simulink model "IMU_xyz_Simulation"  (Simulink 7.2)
settings: Solver=FixedStepDiscrete  StartTime=0.0  StopTime=110  FixedStep=.001  RelTol=1e-3
PreLoadFcn:
  | Script_Kalman
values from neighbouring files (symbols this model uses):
  Az = [1 -Ts ;0 1]    [Script_Kalman.m]
  Kz = 1e-3*[.4 ; -.04]    [Script_Kalman.m]
  Ts = .001    (= 0.001)    [Script_Kalman.m]
undefined symbols (not defined in the file or in its folder): DiscIntNeverNeededParam, float
libraries: simulink x40
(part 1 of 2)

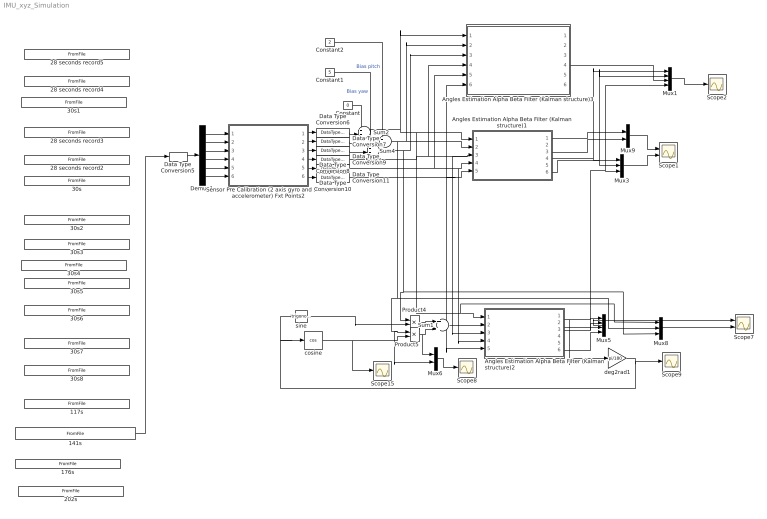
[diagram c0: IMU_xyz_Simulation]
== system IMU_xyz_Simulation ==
  117s : FromFile  FileName=LongLogHorizontalSmallRoll.mat  SampleTime=.001
  141s : FromFile  FileName=LongLongLogHorizontalSmallRoll.mat  SampleTime=.001
  176s : FromFile  FileName=LongLongLogHorizontalSmallRoll2.mat  SampleTime=.001
  202s : FromFile  FileName=LongLongLogHorizontalStatic.mat  SampleTime=.001
  28 seconds record2 : FromFile  FileName=Pitch.mat  SampleTime=.001
  28 seconds record3 : FromFile  FileName=Yaw.mat  SampleTime=.001
  28 seconds record4 : FromFile  FileName=Pitch2.mat  SampleTime=.001
  28 seconds record5 : FromFile  FileName=Yaw2.mat  SampleTime=.001
  30s : FromFile  FileName=Roll.mat  SampleTime=.001
  30s1 : FromFile  FileName=Roll2.mat  SampleTime=.001
  30s2 : FromFile  FileName=Pitch_Up_Calibration.mat  SampleTime=.001
  30s3 : FromFile  FileName=Roll_Right_Calibration.mat  SampleTime=.001
  30s4 : FromFile  FileName=Turn_Left_Roll_Pitch_Yaw.mat  SampleTime=.001
  30s5 : FromFile  FileName=Turn_Left_Right_Roll_Pitch_Yaw.mat  SampleTime=.001
  30s6 : FromFile  FileName=Turn_Left_Right.mat  SampleTime=.001
  30s7 : FromFile  FileName=StaticHorizontal.mat  SampleTime=.001
  30s8 : FromFile  FileName=StaticRoll90.mat  SampleTime=.001
  Angles Estimation Alpha Beta Filter (Kalman structure)1 : Subsystem
  Angles Estimation Alpha Beta Filter (Kalman structure)2 : Subsystem
  Angles Estimation Alpha Beta Filter (Kalman structure)3 : Subsystem
  Constant : Constant  Value=0  OutDataType=sfix(16)  OutScaling=2^0
  Constant1 : Constant  Value=5  OutDataType=sfix(16)  OutScaling=2^0
  Constant2 : Constant  Value=2  OutDataType=sfix(16)  OutScaling=2^0
  Data Type Conversion{6..11} (6 alike) : DataTypeConversion  OutDataType=sfix(16)  OutScaling=2^0
  Data Type Conversion5 : DataTypeConversion  OutDataTypeMode=int16  OutDataType=sfix(16)  OutScaling=2^0  OutDataTypeStr=int16
  Demux1 : Demux  Outputs=6
  Mux1 : Mux
  Mux3 : Mux  Inputs=3
  Mux5 : Mux
  Mux6 : Mux  Inputs=2
  Mux8 : Mux  Inputs=3
  Mux9 : Mux  Inputs=2
  Product4 : Product  OutDataType=sfix(16)  OutScaling=2^0
  Product5 : Product  OutDataType=sfix(16)  OutScaling=2^0
  Scope1 : Scope  NumInputPorts=2
  Scope{2,8..9,15} (4 alike) : Scope
  Scope7 : Scope  NumInputPorts=2
  Sensor Pre Calibration (2 axis gyro and 3 axis accelerometer) Fxt Points2 : Subsystem
  Sum1 : Sum  OutDataType=sfix(16)  OutScaling=2^0
  Sum2 : Sum  Inputs=++|  OutDataType=sfix(16)  OutScaling=2^0
  Sum3 : Sum  Inputs=++|  OutDataType=sfix(16)  OutScaling=2^0
  Sum4 : Sum  Inputs=++|  OutDataType=sfix(16)  OutScaling=2^0
  cosine : Trigonometry  Operator=cos
  deg2rad1 : Gain  Gain=pi/180  ParameterDataType=sfix(16)  ParameterScaling=2^0  OutDataType=sfix(16)  OutScaling=2^0
  sine : Trigonometry
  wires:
  Demux1/1 -> Sensor Pre Calibration (2 axis gyro and 3 axis accelerometer) Fxt Points2/1(Gyro Y)
  Demux1/2 -> Sensor Pre Calibration (2 axis gyro and 3 axis accelerometer) Fxt Points2/2(Accel y)
  Demux1/3 -> Sensor Pre Calibration (2 axis gyro and 3 axis accelerometer) Fxt Points2/3(Accel z)
  Demux1/4 -> Sensor Pre Calibration (2 axis gyro and 3 axis accelerometer) Fxt Points2/4(Gyro X)
  Demux1/5 -> Sensor Pre Calibration (2 axis gyro and 3 axis accelerometer) Fxt Points2/5(Accel x)
  Demux1/6 -> Sensor Pre Calibration (2 axis gyro and 3 axis accelerometer) Fxt Points2/6(Gyro z)
  Data Type Conversion5/1 -> Demux1/1
  Sensor Pre Calibration (2 axis gyro and 3 axis accelerometer) Fxt Points2/6(unbiased Accel Z) -> Data Type Conversion11/1
  Sensor Pre Calibration (2 axis gyro and 3 axis accelerometer) Fxt Points2/1(Gyro Y (degree/s)) -> Data Type Conversion6/1
  Sensor Pre Calibration (2 axis gyro and 3 axis accelerometer) Fxt Points2/2(Gyro X (degree/s)) -> Data Type Conversion7/1
  Sensor Pre Calibration (2 axis gyro and 3 axis accelerometer) Fxt Points2/3(Gyro Z (degree/s)) -> Data Type Conversion8/1
  Data Type Conversion6/1 -> Sum2/2
  Data Type Conversion7/1 -> Sum4/2
  Sensor Pre Calibration (2 axis gyro and 3 axis accelerometer) Fxt Points2/4(unbiased Accel Y) -> Data Type Conversion9/1
  Sensor Pre Calibration (2 axis gyro and 3 axis accelerometer) Fxt Points2/5(unbiased Accel X) -> Data Type Conversion10/1
  Data Type Conversion9/1 -> Angles Estimation Alpha Beta Filter (Kalman structure)3/4(Accel Y), Angles Estimation Alpha Beta Filter (Kalman structure)1/3(Accel Y), Angles Estimation Alpha Beta Filter (Kalman structure)2/3(Accel Y)
  Data Type Conversion10/1 -> Angles Estimation Alpha Beta Filter (Kalman structure)1/4(Accel X), Angles Estimation Alpha Beta Filter (Kalman structure)2/4(Accel X), Angles Estimation Alpha Beta Filter (Kalman structure)3/5(Accel X)
  Data Type Conversion11/1 -> Angles Estimation Alpha Beta Filter (Kalman structure)1/5(Accel Z), Angles Estimation Alpha Beta Filter (Kalman structure)2/5(Accel Z), Angles Estimation Alpha Beta Filter (Kalman structure)3/6(Accel Z)
  Data Type Conversion8/1 -> Sum3/2
  Mux5/1 -> Scope7/1
  Angles Estimation Alpha Beta Filter (Kalman structure)2/1(Angle Estimation Y) -> deg2rad1/1, Mux5/1
  Angles Estimation Alpha Beta Filter (Kalman structure)2/4(Angle Estimation X) -> Mux5/2, Mux3/3, Mux1/4
  deg2rad1/1 -> sine/1, cosine/1, Scope9/1
  cosine/1 -> Product5/2, Scope15/1
  Sum1/1 -> Angles Estimation Alpha Beta Filter (Kalman structure)2/2(Gyro X)
  Product5/1 -> Sum1/2, Mux6/1
  Product4/1 -> Sum1/1
  sine/1 -> Product4/2
  Mux6/1 -> Scope8/1
  Mux8/1 -> Scope7/2
  Angles Estimation Alpha Beta Filter (Kalman structure)2/3(Angle Estimation Y Accel) -> Mux5/3
  Angles Estimation Alpha Beta Filter (Kalman structure)2/6(Angle Estimation X  Accel) -> Mux5/4
  Angles Estimation Alpha Beta Filter (Kalman structure)1/1(Angle Estimation Y) -> Mux9/1
  Angles Estimation Alpha Beta Filter (Kalman structure)1/3(Angle Estimation Y Accel) -> Mux9/2
  Angles Estimation Alpha Beta Filter (Kalman structure)1/4(Angle Estimation X) -> Mux3/1, Mux1/1
  Angles Estimation Alpha Beta Filter (Kalman structure)1/6(Angle Estimation X  Accel) -> Mux3/2, Mux1/2
  Mux9/1 -> Scope1/1
  Mux3/1 -> Scope1/2
  Angles Estimation Alpha Beta Filter (Kalman structure)3/4(Angle Estimation X) -> Mux1/3
  Mux1/1 -> Scope2/1
  Sum2/1 -> Angles Estimation Alpha Beta Filter (Kalman structure)2/1(Gyro Y), Mux8/1, Angles Estimation Alpha Beta Filter (Kalman structure)1/1(Gyro Y), Angles Estimation Alpha Beta Filter (Kalman structure)3/1(Gyro Y)
  Constant/1 -> Sum2/1
  Sum3/1 -> Angles Estimation Alpha Beta Filter (Kalman structure)3/3(Gyro Z), Product4/1, Mux8/3
  Constant1/1 -> Sum3/1  "Bias yaw"
  Sum4/1 -> Product5/1, Mux6/2, Mux8/2, Angles Estimation Alpha Beta Filter (Kalman structure)3/2(Gyro X), Angles Estimation Alpha Beta Filter (Kalman structure)1/2(Gyro X)
  Constant2/1 -> Sum4/1  "Bias pitch"
  141s/1 -> Data Type Conversion5/1

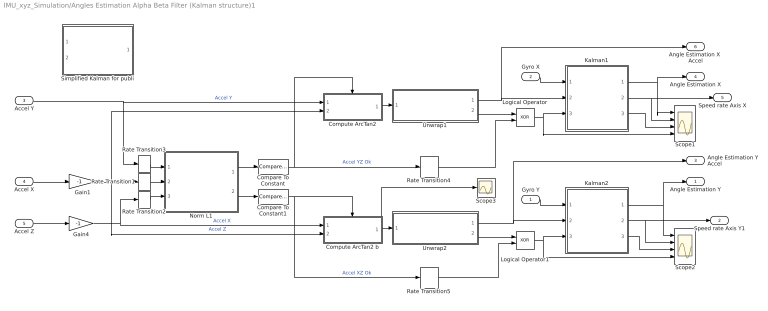
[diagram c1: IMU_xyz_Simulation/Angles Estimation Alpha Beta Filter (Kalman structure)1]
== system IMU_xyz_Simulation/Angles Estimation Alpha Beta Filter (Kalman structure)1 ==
  Gyro Y : Inport
  Gyro X : Inport  Port=2
  Accel Y : Inport  Port=3
  Accel X : Inport  Port=4
  Accel Z : Inport  Port=5
  Compare To Constant : simulink/Logic and Bit Operations/Compare To Constant  SystemSampleTime=-1  relop=>=  const=200  LogicOutDataTypeMode=boolean  ZeroCross=off
  Compare To Constant1 : simulink/Logic and Bit Operations/Compare To Constant  SystemSampleTime=-1  relop=>=  const=200  LogicOutDataTypeMode=boolean  ZeroCross=off
  Compute ArcTan2 : Subsystem
  Compute ArcTan2 b : Subsystem
  Gain1 : Gain  Gain=-1  ParameterDataType=sfix(16)  ParameterScaling=2^0  OutDataType=sfix(16)  OutScaling=2^0
  Gain4 : Gain  Gain=-1  ParameterDataType=sfix(16)  ParameterScaling=2^0  OutDataType=sfix(16)  OutScaling=2^0
  Kalman1 : Subsystem
  Kalman2 : Subsystem
  Logical Operator : Logic  Operator=XOR  AllPortsSameDT=off  OutDataTypeMode=boolean  OutDataTypeStr=boolean
  Logical Operator1 : Logic  Operator=XOR  AllPortsSameDT=off  OutDataTypeMode=boolean  OutDataTypeStr=boolean
  Norm L1 : Subsystem
  Rate Transition1 : RateTransition  Integrity=off  OutPortSampleTime=.2
  Rate Transition2 : RateTransition  Integrity=off  OutPortSampleTime=.2
  Rate Transition3 : RateTransition  Integrity=off  OutPortSampleTime=.2
  Rate Transition4 : RateTransition  Integrity=off  OutPortSampleTime=.001
  Rate Transition5 : RateTransition  Integrity=off  OutPortSampleTime=.001
  Scope1 : Scope  NumInputPorts=4
  Scope2 : Scope  NumInputPorts=4
  Scope3 : Scope
  Simplified Kalman for publi : Subsystem
  Unwrap1 : Subsystem
  Unwrap2 : Subsystem
  Angle Estimation Y : Outport
  Speed rate Axis Y1 : Outport  Port=2
  Angle Estimation Y Accel : Outport  Port=3
  Angle Estimation X : Outport  Port=4
  Speed rate Axis X : Outport  Port=5
  Angle Estimation X  Accel : Outport  Port=6
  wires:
  Kalman1/3(Bias) -> Scope1/3
  Kalman2/3(Bias) -> Scope2/3
  Kalman2/2(Speed) -> Speed rate Axis Y1/1, Scope2/2
  Kalman1/2(Speed) -> Speed rate Axis X/1, Scope1/2
  Unwrap2/1(unwrap angle) -> Angle Estimation Y Accel/1, Kalman2/2(Accel1)
  Unwrap2/2(Wrap) -> Logical Operator1/1
  Logical Operator/1 -> Scope1/4, Kalman1/3(Adapt1)
  Rate Transition5/1 -> Logical Operator1/2
  Gain1/1 -> Compute ArcTan2 b/2(Force 2), Rate Transition1/1, Compute ArcTan2/2(Force 2)  "Accel Z"
  Logical Operator1/1 -> Kalman2/3(Adapt1), Scope2/4
  Rate Transition4/1 -> Logical Operator/2
  Unwrap1/2(Wrap) -> Logical Operator/1
  Unwrap1/1(unwrap angle) -> Angle Estimation X  Accel/1, Kalman1/2(Accel1)
  Rate Transition3/1 -> Norm L1/1(Accel Y)
  Rate Transition2/1 -> Norm L1/3(Accel X)
  Rate Transition1/1 -> Norm L1/2(Accel Z)
  Kalman2/1(Position) -> Scope2/1, Angle Estimation Y/1
  Kalman1/1(Position) -> Scope1/1, Angle Estimation X/1
  Compare To Constant1/1 -> Rate Transition5/1, Compute ArcTan2 b/Enable  "Accel XZ Ok"
  Compare To Constant/1 -> Rate Transition4/1, Compute ArcTan2/Enable  "Accel YZ Ok"
  Norm L1/1(abs(Y)+abs(Z)) -> Compare To Constant/1
  Norm L1/2(abs(X)+abs(Z)) -> Compare To Constant1/1
  Accel X/1 -> Gain1/1
  Gain4/1 -> Compute ArcTan2 b/1(Force 1), Rate Transition2/1  "Accel X"
  Compute ArcTan2/1(Degree) -> Unwrap1/1(Estimated Angle)
  Compute ArcTan2 b/1(Degree) -> Scope3/1, Unwrap2/1(Estimated Angle)
  Accel Z/1 -> Gain4/1
  Accel Y/1 -> Compute ArcTan2/1(Force 1), Rate Transition3/1  "Accel Y"
  Gyro X/1 -> Kalman1/1(Gyro)
  Gyro Y/1 -> Kalman2/1(Gyro)

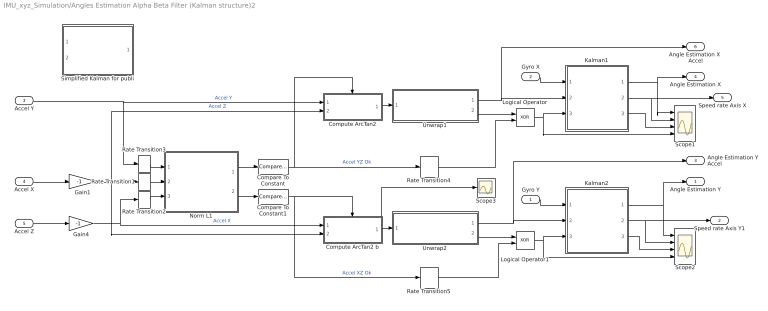
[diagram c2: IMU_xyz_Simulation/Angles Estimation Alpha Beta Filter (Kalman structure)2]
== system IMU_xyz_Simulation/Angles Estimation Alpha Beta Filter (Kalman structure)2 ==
  Gyro Y : Inport
  Gyro X : Inport  Port=2
  Accel Y : Inport  Port=3
  Accel X : Inport  Port=4
  Accel Z : Inport  Port=5
  Compare To Constant : simulink/Logic and Bit Operations/Compare To Constant  SystemSampleTime=-1  relop=>=  const=200  LogicOutDataTypeMode=boolean  ZeroCross=off
  Compare To Constant1 : simulink/Logic and Bit Operations/Compare To Constant  SystemSampleTime=-1  relop=>=  const=200  LogicOutDataTypeMode=boolean  ZeroCross=off
  Compute ArcTan2 : Subsystem
  Compute ArcTan2 b : Subsystem
  Gain1 : Gain  Gain=-1  ParameterDataType=sfix(16)  ParameterScaling=2^0  OutDataType=sfix(16)  OutScaling=2^0
  Gain4 : Gain  Gain=-1  ParameterDataType=sfix(16)  ParameterScaling=2^0  OutDataType=sfix(16)  OutScaling=2^0
  Kalman1 : Subsystem
  Kalman2 : Subsystem
  Logical Operator : Logic  Operator=XOR  AllPortsSameDT=off  OutDataTypeMode=boolean  OutDataTypeStr=boolean
  Logical Operator1 : Logic  Operator=XOR  AllPortsSameDT=off  OutDataTypeMode=boolean  OutDataTypeStr=boolean
  Norm L1 : Subsystem
  Rate Transition1 : RateTransition  Integrity=off  OutPortSampleTime=.2
  Rate Transition2 : RateTransition  Integrity=off  OutPortSampleTime=.2
  Rate Transition3 : RateTransition  Integrity=off  OutPortSampleTime=.2
  Rate Transition4 : RateTransition  Integrity=off  OutPortSampleTime=.001
  Rate Transition5 : RateTransition  Integrity=off  OutPortSampleTime=.001
  Scope1 : Scope  NumInputPorts=4
  Scope2 : Scope  NumInputPorts=4
  Scope3 : Scope
  Simplified Kalman for publi : Subsystem
  Unwrap1 : Subsystem
  Unwrap2 : Subsystem
  Angle Estimation Y : Outport
  Speed rate Axis Y1 : Outport  Port=2
  Angle Estimation Y Accel : Outport  Port=3
  Angle Estimation X : Outport  Port=4
  Speed rate Axis X : Outport  Port=5
  Angle Estimation X  Accel : Outport  Port=6
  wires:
  Gyro Y/1 -> Kalman2/1(Gyro)
  Gyro X/1 -> Kalman1/1(Gyro)
  Accel Y/1 -> Rate Transition3/1, Compute ArcTan2/1(Force 1)  "Accel Y"
  Accel Z/1 -> Gain4/1
  Compute ArcTan2 b/1(Degree) -> Unwrap2/1(Estimated Angle), Scope3/1
  Compute ArcTan2/1(Degree) -> Unwrap1/1(Estimated Angle)
  Gain4/1 -> Rate Transition2/1, Compute ArcTan2 b/1(Force 1)  "Accel X"
  Accel X/1 -> Gain1/1
  Norm L1/2(abs(X)+abs(Z)) -> Compare To Constant1/1
  Norm L1/1(abs(Y)+abs(Z)) -> Compare To Constant/1
  Compare To Constant/1 -> Compute ArcTan2/Enable, Rate Transition4/1  "Accel YZ Ok"
  Compare To Constant1/1 -> Compute ArcTan2 b/Enable, Rate Transition5/1  "Accel XZ Ok"
  Kalman1/1(Position) -> Angle Estimation X/1, Scope1/1
  Kalman2/1(Position) -> Angle Estimation Y/1, Scope2/1
  Rate Transition1/1 -> Norm L1/2(Accel Z)
  Rate Transition2/1 -> Norm L1/3(Accel X)
  Rate Transition3/1 -> Norm L1/1(Accel Y)
  Unwrap1/1(unwrap angle) -> Kalman1/2(Accel1), Angle Estimation X  Accel/1
  Unwrap1/2(Wrap) -> Logical Operator/1
  Rate Transition4/1 -> Logical Operator/2
  Logical Operator1/1 -> Scope2/4, Kalman2/3(Adapt1)
  Gain1/1 -> Compute ArcTan2/2(Force 2), Rate Transition1/1, Compute ArcTan2 b/2(Force 2)  "Accel Z"
  Rate Transition5/1 -> Logical Operator1/2
  Logical Operator/1 -> Kalman1/3(Adapt1), Scope1/4
  Unwrap2/2(Wrap) -> Logical Operator1/1
  Unwrap2/1(unwrap angle) -> Kalman2/2(Accel1), Angle Estimation Y Accel/1
  Kalman1/2(Speed) -> Scope1/2, Speed rate Axis X/1
  Kalman2/2(Speed) -> Scope2/2, Speed rate Axis Y1/1
  Kalman2/3(Bias) -> Scope2/3
  Kalman1/3(Bias) -> Scope1/3

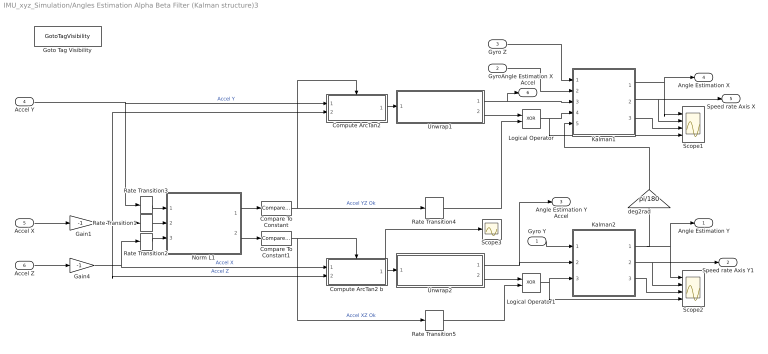
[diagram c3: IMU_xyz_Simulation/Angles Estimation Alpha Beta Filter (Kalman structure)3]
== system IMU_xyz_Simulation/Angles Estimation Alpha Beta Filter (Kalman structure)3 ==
  Gyro Y : Inport
  Gyro X : Inport  Port=2
  Gyro Z : Inport  Port=3
  Accel Y : Inport  Port=4
  Accel X : Inport  Port=5
  Accel Z : Inport  Port=6
  Compare To Constant : simulink/Logic and Bit Operations/Compare To Constant  SystemSampleTime=-1  relop=>=  const=200  LogicOutDataTypeMode=boolean  ZeroCross=off
  Compare To Constant1 : simulink/Logic and Bit Operations/Compare To Constant  SystemSampleTime=-1  relop=>=  const=200  LogicOutDataTypeMode=boolean  ZeroCross=off
  Compute ArcTan2 : Subsystem
  Compute ArcTan2 b : Subsystem
  Gain1 : Gain  Gain=-1  ParameterDataType=sfix(16)  ParameterScaling=2^0  OutDataType=sfix(16)  OutScaling=2^0
  Gain4 : Gain  Gain=-1  ParameterDataType=sfix(16)  ParameterScaling=2^0  OutDataType=sfix(16)  OutScaling=2^0
  Goto Tag Visibility : GotoTagVisibility
  Kalman1 : Subsystem
  Kalman2 : Subsystem
  Logical Operator : Logic  Operator=XOR  AllPortsSameDT=off  OutDataTypeMode=boolean  OutDataTypeStr=boolean
  Logical Operator1 : Logic  Operator=XOR  AllPortsSameDT=off  OutDataTypeMode=boolean  OutDataTypeStr=boolean
  Norm L1 : Subsystem
  Rate Transition1 : RateTransition  Integrity=off  OutPortSampleTime=.2
  Rate Transition2 : RateTransition  Integrity=off  OutPortSampleTime=.2
  Rate Transition3 : RateTransition  Integrity=off  OutPortSampleTime=.2
  Rate Transition4 : RateTransition  Integrity=off  OutPortSampleTime=.001
  Rate Transition5 : RateTransition  Integrity=off  OutPortSampleTime=.001
  Scope1 : Scope  NumInputPorts=4
  Scope2 : Scope  NumInputPorts=4
  Scope3 : Scope
  Unwrap1 : Subsystem
  Unwrap2 : Subsystem
  deg2rad : Gain  Orientation=up  Gain=pi/180  ParameterDataType=sfix(16)  ParameterScaling=2^0  OutDataType=sfix(16)  OutScaling=2^0
  Angle Estimation Y : Outport
  Speed rate Axis Y1 : Outport  Port=2
  Angle Estimation Y Accel : Outport  Port=3
  Angle Estimation X : Outport  Port=4
  Speed rate Axis X : Outport  Port=5
  Angle Estimation X  Accel : Outport  Port=6
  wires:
  Kalman1/3(Bias) -> Scope1/3
  Kalman2/3(Bias) -> Scope2/3
  Kalman2/2(Speed) -> Speed rate Axis Y1/1, Scope2/2
  Kalman1/2(Speed) -> Speed rate Axis X/1, Scope1/2
  Unwrap2/1(unwrap angle) -> Angle Estimation Y Accel/1, Kalman2/2(Accel1)
  Unwrap2/2(Wrap) -> Logical Operator1/1
  Logical Operator/1 -> Scope1/4, Kalman1/4(Adapt1)
  Rate Transition5/1 -> Logical Operator1/2
  Gain1/1 -> Compute ArcTan2 b/2(Force 2), Rate Transition1/1, Compute ArcTan2/2(Force 2)  "Accel Z"
  Logical Operator1/1 -> Kalman2/3(Adapt1), Scope2/4
  Rate Transition4/1 -> Logical Operator/2
  Unwrap1/2(Wrap) -> Logical Operator/1
  Unwrap1/1(unwrap angle) -> Angle Estimation X  Accel/1, Kalman1/3(Accel1)
  Rate Transition3/1 -> Norm L1/1(Accel Y)
  Rate Transition2/1 -> Norm L1/3(Accel X)
  Rate Transition1/1 -> Norm L1/2(Accel Z)
  Kalman2/1(Position) -> Scope2/1, Angle Estimation Y/1, deg2rad/1
  Kalman1/1(Position) -> Scope1/1, Angle Estimation X/1
  Compare To Constant1/1 -> Rate Transition5/1, Compute ArcTan2 b/Enable  "Accel XZ Ok"
  Compare To Constant/1 -> Rate Transition4/1, Compute ArcTan2/Enable  "Accel YZ Ok"
  Norm L1/1(abs(Y)+abs(Z)) -> Compare To Constant/1
  Norm L1/2(abs(X)+abs(Z)) -> Compare To Constant1/1
  Accel X/1 -> Gain1/1
  Gain4/1 -> Compute ArcTan2 b/1(Force 1), Rate Transition2/1  "Accel X"
  Compute ArcTan2/1(Degree) -> Unwrap1/1(Estimated Angle)
  Compute ArcTan2 b/1(Degree) -> Scope3/1, Unwrap2/1(Estimated Angle)
  Accel Z/1 -> Gain4/1
  Accel Y/1 -> Compute ArcTan2/1(Force 1), Rate Transition3/1  "Accel Y"
  Gyro Y/1 -> Kalman2/1(Gyro)
  Gyro X/1 -> Kalman1/2(Gyro X1)
  Gyro Z/1 -> Kalman1/1(Gyro Z)
  deg2rad/1 -> Kalman1/5(Roll Angle (rad))

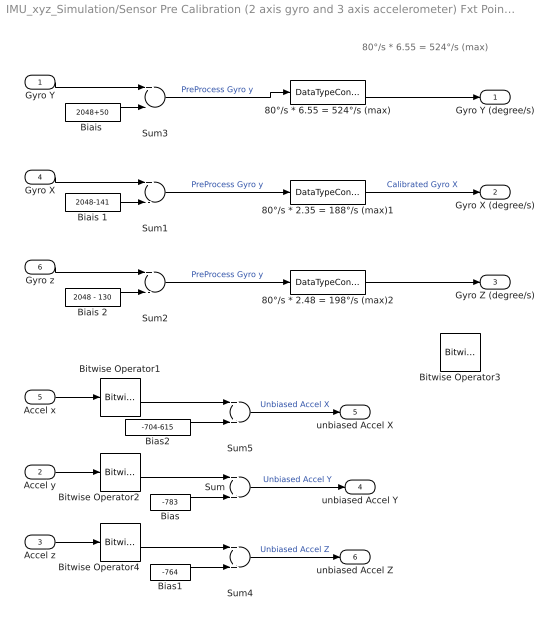
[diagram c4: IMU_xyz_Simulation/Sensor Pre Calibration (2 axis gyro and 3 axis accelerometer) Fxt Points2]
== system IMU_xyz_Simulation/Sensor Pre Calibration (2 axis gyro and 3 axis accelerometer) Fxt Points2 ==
  note: 80°/s * 6.55 = 524°/s (max)
  Gyro Y : Inport
  Accel y : Inport  Port=2
  Accel z : Inport  Port=3
  Gyro X : Inport  Port=4
  Accel x : Inport  Port=5
  Gyro z : Inport  Port=6
  80°/s * 2.35 = 188°/s (max)1 : DataTypeConversion  OutDataTypeMode=Specify via dialog  OutDataType=fixdt(1,16,80/2048*2.49,0)  OutDataTypeStr=fixdt(1,16,80/2048*2.49,0)  ConvertRealWorld=Stored Integer (SI)
  80°/s * 2.48 = 198°/s (max)2 : DataTypeConversion  OutDataTypeMode=Specify via dialog  OutDataType=fixdt(1,16,80/2048*2.5,0)  OutDataTypeStr=fixdt(1,16,80/2048*2.5,0)  ConvertRealWorld=Stored Integer (SI)
  80°/s * 6.55 = 524°/s (max) : DataTypeConversion  OutDataTypeMode=Specify via dialog  OutDataType=fixdt(1,16,80/2048*4.93,0)  OutDataTypeStr=fixdt(1,16,80/2048*4.93,0)  ConvertRealWorld=Stored Integer (SI)
  "Biais " : Constant  Value=2048+50  OutDataType=sfix(16)  OutScaling=2^0  OutDataTypeStr=Inherit: Inherit via back propagation
  Biais 1 : Constant  Value=2048-141  OutDataType=sfix(16)  OutScaling=2^0  OutDataTypeStr=Inherit: Inherit via back propagation
  Biais 2 : Constant  Value=2048 - 130  OutDataType=sfix(16)  OutScaling=2^0  OutDataTypeStr=Inherit: Inherit via back propagation
  Bias : Constant  Value=-783  OutDataType=sfix(16)  OutScaling=2^0  OutDataTypeStr=Inherit: Inherit via back propagation
  Bias1 : Constant  Value=-764  OutDataType=sfix(16)  OutScaling=2^0  OutDataTypeStr=Inherit: Inherit via back propagation
  Bias2 : Constant  Value=-704-615  OutDataType=sfix(16)  OutScaling=2^0  OutDataTypeStr=Inherit: Inherit via back propagation
  Bitwise Operator{1..4} (4 alike) : simulink/Logic and Bit Operations/Bitwise Operator  logicop=AND  UseBitMask=on  BitMask=4095  BitMaskRealWorld=Stored Integer
  Sum : Sum  OutDataTypeMode=int16  OutDataType=sfix(16)  OutScaling=2^0  OutDataTypeStr=int16
  Sum1 : Sum  Inputs=+-  OutDataTypeMode=int16  OutDataType=sfix(16)  OutScaling=2^0  OutDataTypeStr=int16
  Sum2 : Sum  Inputs=+-  OutDataTypeMode=int16  OutDataType=sfix(16)  OutScaling=2^0  OutDataTypeStr=int16
  Sum3 : Sum  Inputs=+-  OutDataTypeMode=int16  OutDataType=sfix(16)  OutScaling=2^0  OutDataTypeStr=int16
  Sum4 : Sum  OutDataTypeMode=int16  OutDataType=sfix(16)  OutScaling=2^0  OutDataTypeStr=int16
  Sum5 : Sum  OutDataTypeMode=int16  OutDataType=sfix(16)  OutScaling=2^0  OutDataTypeStr=int16
  Gyro Y (degree/s) : Outport
  Gyro X (degree/s) : Outport  Port=2
  Gyro Z (degree/s) : Outport  Port=3
  unbiased Accel Y : Outport  Port=4
  unbiased Accel X : Outport  Port=5
  unbiased Accel Z : Outport  Port=6
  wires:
  Gyro X/1 -> Sum1/1
  Biais 1/1 -> Sum1/2
  Gyro Y/1 -> Sum3/1
  "Biais "/1 -> Sum3/2
  Gyro z/1 -> Sum2/1
  Biais 2/1 -> Sum2/2
  Accel z/1 -> Bitwise Operator4/1
  Accel y/1 -> Bitwise Operator2/1
  Sum3/1 -> 80°/s * 6.55 = 524°/s (max)/1  "PreProcess Gyro y"
  Sum2/1 -> 80°/s * 2.48 = 198°/s (max)2/1  "PreProcess Gyro y"
  Bias/1 -> Sum/2
  Bias1/1 -> Sum4/2
  Bias2/1 -> Sum5/2
  Sum/1 -> unbiased Accel Y/1  "Unbiased Accel Y"
  Sum4/1 -> unbiased Accel Z/1  "Unbiased Accel Z"
  Sum5/1 -> unbiased Accel X/1  "Unbiased Accel X"
  80°/s * 6.55 = 524°/s (max)/1 -> Gyro Y (degree/s)/1
  80°/s * 2.35 = 188°/s (max)1/1 -> Gyro X (degree/s)/1  "Calibrated Gyro X"
  80°/s * 2.48 = 198°/s (max)2/1 -> Gyro Z (degree/s)/1
  Sum1/1 -> 80°/s * 2.35 = 188°/s (max)1/1  "PreProcess Gyro y"
  Accel x/1 -> Bitwise Operator1/1
  Bitwise Operator1/1 -> Sum5/1
  Bitwise Operator2/1 -> Sum/1
  Bitwise Operator4/1 -> Sum4/1

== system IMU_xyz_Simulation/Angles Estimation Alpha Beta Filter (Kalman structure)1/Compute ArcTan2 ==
  Force 1 : Inport
  Force 2 : Inport  Port=2
  Enable : EnablePort  StatesWhenEnabling=reset
  Gain1 : Gain  Gain=180/pi  ParameterDataType=sfix(16)  ParameterScaling=2^0  OutDataTypeMode=Specify via dialog  OutDataType=float('double')  OutDataTypeStr=float('double')
  Trigonometric Function1 : Trigonometry  Operator=atan2  OutputSignalType=real
  Degree : Outport
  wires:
  Force 2/1 -> Trigonometric Function1/2
  Force 1/1 -> Trigonometric Function1/1
  Gain1/1 -> Degree/1
  Trigonometric Function1/1 -> Gain1/1

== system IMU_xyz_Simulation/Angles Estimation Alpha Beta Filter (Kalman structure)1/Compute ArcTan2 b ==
  Force 1 : Inport
  Force 2 : Inport  Port=2
  Enable : EnablePort  StatesWhenEnabling=reset
  Gain1 : Gain  Gain=180/pi  ParameterDataType=sfix(16)  ParameterScaling=2^0  OutDataTypeMode=Specify via dialog  OutDataType=float('double')  OutDataTypeStr=float('double')
  Trigonometric Function1 : Trigonometry  Operator=atan2  OutputSignalType=real
  Degree : Outport
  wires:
  Trigonometric Function1/1 -> Gain1/1
  Gain1/1 -> Degree/1
  Force 1/1 -> Trigonometric Function1/1
  Force 2/1 -> Trigonometric Function1/2

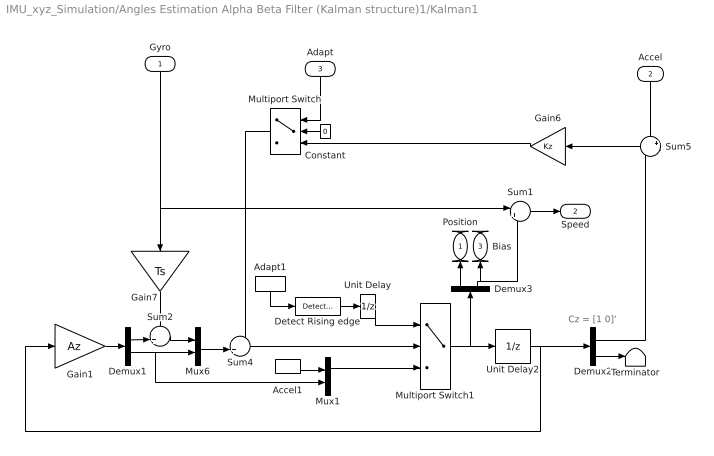
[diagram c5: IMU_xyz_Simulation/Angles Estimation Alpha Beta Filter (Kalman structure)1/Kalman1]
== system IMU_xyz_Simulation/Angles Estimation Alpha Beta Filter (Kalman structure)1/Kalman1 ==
  note: Cz = [1 0]'
  Gyro : Inport  Orientation=down
  Accel : Inport  Orientation=down  Port=2
  Adapt : Inport  Orientation=down  Port=3
  Accel1 : InportShadow  Port=2  LatchByCopyingInsideSignal=off
  Adapt1 : InportShadow  Orientation=down  Port=3  LatchByCopyingInsideSignal=off
  Constant : Constant  Orientation=left  Value=0  OutDataType=sfix(16)  OutScaling=2^0
  Demux1 : Demux  Outputs=2
  Demux2 : Demux  Outputs=2
  Demux3 : Demux  Orientation=up  Outputs=2
  Detect Rising edge : simulink/Logic and Bit Operations/Detect Increase  SystemSampleTime=-1  vinit=0
  Gain1 : Gain  Gain=Az  Multiplication=Matrix(K*u)  ParameterDataType=sfix(16)  ParameterScaling=2^0  OutDataType=sfix(16)  OutScaling=2^0
  Gain6 : Gain  Orientation=left  Gain=Kz  Multiplication=Matrix(K*u)  ParameterDataType=sfix(16)  ParameterScaling=2^0  OutDataType=sfix(16)  OutScaling=2^0
  Gain7 : Gain  Orientation=down  Gain=Ts  Multiplication=Matrix(K*u)  ParameterDataType=sfix(16)  ParameterScaling=2^0  OutDataType=sfix(16)  OutScaling=2^0
  Multiport Switch : MultiPortSwitch  Orientation=left  Inputs=2  zeroidx=on
  Multiport Switch1 : MultiPortSwitch  Inputs=2  zeroidx=on
  Mux1 : Mux  Inputs=2
  Mux6 : Mux  Inputs=2
  Sum1 : Sum  Inputs=|+-  OutDataType=sfix(16)  OutScaling=2^0
  Sum2 : Sum  Inputs=++|  OutDataType=sfix(16)  OutScaling=2^0
  Sum4 : Sum  Inputs=++|  OutDataType=sfix(16)  OutScaling=2^0
  Sum5 : Sum  Orientation=left  Inputs=+-  OutDataType=sfix(16)  OutScaling=2^0
  Terminator : Terminator
  Unit Delay : UnitDelay  SampleTime=-1
  Unit Delay2 : UnitDelay  SampleTime=-1
  Position : Outport  Orientation=up  OutDataType=sfix(16)  OutScaling=2^0
  Speed : Outport  Port=2  OutDataType=sfix(16)  OutScaling=2^0
  Bias : Outport  Orientation=up  Port=3  OutDataType=sfix(16)  OutScaling=2^0
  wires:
  Demux2/2 -> Terminator/1
  Mux1/1 -> Multiport Switch1/3
  Accel1/1 -> Mux1/1
  Adapt1/1 -> Detect Rising edge/1
  Sum4/1 -> Multiport Switch1/2
  Multiport Switch1/1 -> Unit Delay2/1, Demux3/1
  Detect Rising edge/1 -> Unit Delay/1
  Constant/1 -> Multiport Switch/2
  Gain6/1 -> Multiport Switch/3
  Adapt/1 -> Multiport Switch/1
  Multiport Switch/1 -> Sum4/1
  Demux2/1 -> Sum5/2
  Gain1/1 -> Demux1/1
  Demux1/1 -> Sum2/2
  Sum2/1 -> Mux6/1
  Demux1/2 -> Mux1/2, Mux6/2
  Mux6/1 -> Sum4/2
  Sum5/1 -> Gain6/1
  Gain7/1 -> Sum2/1
  Accel/1 -> Sum5/1
  Gyro/1 -> Gain7/1, Sum1/1
  Unit Delay/1 -> Multiport Switch1/1
  Unit Delay2/1 -> Demux2/1, Gain1/1
  Demux3/1 -> Position/1
  Demux3/2 -> Bias/1, Sum1/2
  Sum1/1 -> Speed/1

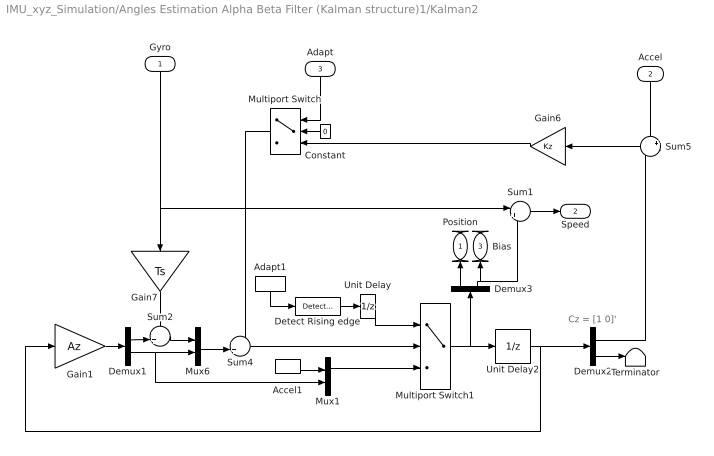
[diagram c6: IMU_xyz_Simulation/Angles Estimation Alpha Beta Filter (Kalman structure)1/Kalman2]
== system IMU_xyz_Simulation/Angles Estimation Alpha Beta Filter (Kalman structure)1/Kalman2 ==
  note: Cz = [1 0]'
  Gyro : Inport  Orientation=down
  Accel : Inport  Orientation=down  Port=2
  Adapt : Inport  Orientation=down  Port=3
  Accel1 : InportShadow  Port=2  LatchByCopyingInsideSignal=off
  Adapt1 : InportShadow  Orientation=down  Port=3  LatchByCopyingInsideSignal=off
  Constant : Constant  Orientation=left  Value=0  OutDataType=sfix(16)  OutScaling=2^0
  Demux1 : Demux  Outputs=2
  Demux2 : Demux  Outputs=2
  Demux3 : Demux  Orientation=up  Outputs=2
  Detect Rising edge : simulink/Logic and Bit Operations/Detect Increase  SystemSampleTime=-1  vinit=0
  Gain1 : Gain  Gain=Az  Multiplication=Matrix(K*u)  ParameterDataType=sfix(16)  ParameterScaling=2^0  OutDataType=sfix(16)  OutScaling=2^0
  Gain6 : Gain  Orientation=left  Gain=Kz  Multiplication=Matrix(K*u)  ParameterDataType=sfix(16)  ParameterScaling=2^0  OutDataType=sfix(16)  OutScaling=2^0
  Gain7 : Gain  Orientation=down  Gain=Ts  Multiplication=Matrix(K*u)  ParameterDataType=sfix(16)  ParameterScaling=2^0  OutDataType=sfix(16)  OutScaling=2^0
  Multiport Switch : MultiPortSwitch  Orientation=left  Inputs=2  zeroidx=on
  Multiport Switch1 : MultiPortSwitch  Inputs=2  zeroidx=on
  Mux1 : Mux  Inputs=2
  Mux6 : Mux  Inputs=2
  Sum1 : Sum  Inputs=|+-  OutDataType=sfix(16)  OutScaling=2^0
  Sum2 : Sum  Inputs=++|  OutDataType=sfix(16)  OutScaling=2^0
  Sum4 : Sum  Inputs=++|  OutDataType=sfix(16)  OutScaling=2^0
  Sum5 : Sum  Orientation=left  Inputs=+-  OutDataType=sfix(16)  OutScaling=2^0
  Terminator : Terminator
  Unit Delay : UnitDelay  SampleTime=-1
  Unit Delay2 : UnitDelay  SampleTime=-1
  Position : Outport  Orientation=up  OutDataType=sfix(16)  OutScaling=2^0
  Speed : Outport  Port=2  OutDataType=sfix(16)  OutScaling=2^0
  Bias : Outport  Orientation=up  Port=3  OutDataType=sfix(16)  OutScaling=2^0
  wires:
  Sum1/1 -> Speed/1
  Demux3/2 -> Sum1/2, Bias/1
  Demux3/1 -> Position/1
  Unit Delay2/1 -> Gain1/1, Demux2/1
  Unit Delay/1 -> Multiport Switch1/1
  Gyro/1 -> Sum1/1, Gain7/1
  Accel/1 -> Sum5/1
  Gain7/1 -> Sum2/1
  Sum5/1 -> Gain6/1
  Mux6/1 -> Sum4/2
  Demux1/2 -> Mux6/2, Mux1/2
  Sum2/1 -> Mux6/1
  Demux1/1 -> Sum2/2
  Gain1/1 -> Demux1/1
  Demux2/1 -> Sum5/2
  Multiport Switch/1 -> Sum4/1
  Adapt/1 -> Multiport Switch/1
  Gain6/1 -> Multiport Switch/3
  Constant/1 -> Multiport Switch/2
  Detect Rising edge/1 -> Unit Delay/1
  Multiport Switch1/1 -> Demux3/1, Unit Delay2/1
  Sum4/1 -> Multiport Switch1/2
  Adapt1/1 -> Detect Rising edge/1
  Accel1/1 -> Mux1/1
  Mux1/1 -> Multiport Switch1/3
  Demux2/2 -> Terminator/1

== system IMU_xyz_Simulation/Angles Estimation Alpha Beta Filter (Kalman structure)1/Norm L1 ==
  Accel Y : Inport
  Accel Z : Inport  Port=2
  Accel X : Inport  Port=3
  Abs : Abs
  Abs1 : Abs
  Abs2 : Abs
  Sum1 : Sum  OutDataType=sfix(16)  OutScaling=2^0
  Sum3 : Sum  OutDataType=sfix(16)  OutScaling=2^0
  abs(Y)+abs(Z) : Outport
  abs(X)+abs(Z) : Outport  Port=2
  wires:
  Sum1/1 -> abs(X)+abs(Z)/1
  Accel X/1 -> Abs2/1
  Abs2/1 -> Sum1/2
  Sum3/1 -> abs(Y)+abs(Z)/1
  Accel Z/1 -> Abs1/1
  Accel Y/1 -> Abs/1
  Abs1/1 -> Sum3/2, Sum1/1
  Abs/1 -> Sum3/1

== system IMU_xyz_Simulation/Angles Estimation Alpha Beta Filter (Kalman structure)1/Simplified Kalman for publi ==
  note: Cz = [1 0]'
  Gyro : Inport  Orientation=down
  Accel : Inport  Orientation=down  Port=2
  Demux1 : Demux  Outputs=2
  Demux2 : Demux  Outputs=2
  Gain1 : Gain  Gain=Az  Multiplication=Matrix(K*u)  ParameterDataType=sfix(16)  ParameterScaling=2^0  OutDataType=sfix(16)  OutScaling=2^0
  Gain6 : Gain  Orientation=left  Gain=Kz  Multiplication=Matrix(K*u)  ParameterDataType=sfix(16)  ParameterScaling=2^0  OutDataType=sfix(16)  OutScaling=2^0
  Gain7 : Gain  Orientation=down  Gain=Ts  Multiplication=Matrix(K*u)  ParameterDataType=sfix(16)  ParameterScaling=2^0  OutDataType=sfix(16)  OutScaling=2^0
  Mux6 : Mux  Inputs=2
  Sum2 : Sum  Inputs=++|  OutDataType=sfix(16)  OutScaling=2^0
  Sum4 : Sum  Inputs=++|  OutDataType=sfix(16)  OutScaling=2^0
  Sum5 : Sum  Orientation=left  Inputs=+-  OutDataType=sfix(16)  OutScaling=2^0
  Terminator : Terminator
  Unit Delay2 : UnitDelay  SampleTime=-1
  Angle Estimation : Outport  OutDataType=sfix(16)  OutScaling=2^0
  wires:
  Gain6/1 -> Sum4/1
  Unit Delay2/1 -> Gain1/1, Demux2/1
  Gyro/1 -> Gain7/1
  Accel/1 -> Sum5/1
  Gain7/1 -> Sum2/1
  Sum5/1 -> Gain6/1
  Mux6/1 -> Sum4/2
  Demux1/2 -> Mux6/2  "Gyro Bias"
  Sum2/1 -> Mux6/1  "Angle Estimation"
  Demux1/1 -> Sum2/2
  Gain1/1 -> Demux1/1
  Demux2/1 -> Angle Estimation/1, Sum5/2
  Sum4/1 -> Unit Delay2/1
  Demux2/2 -> Terminator/1

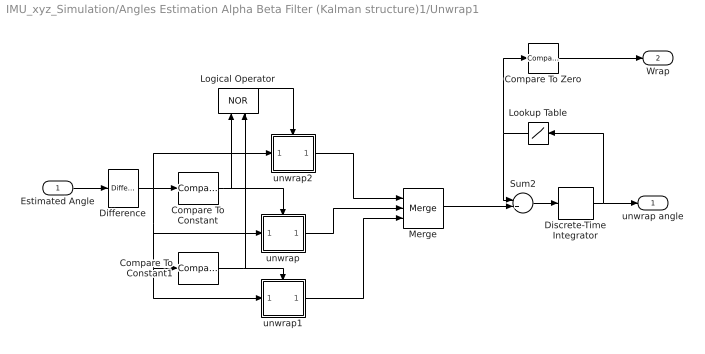
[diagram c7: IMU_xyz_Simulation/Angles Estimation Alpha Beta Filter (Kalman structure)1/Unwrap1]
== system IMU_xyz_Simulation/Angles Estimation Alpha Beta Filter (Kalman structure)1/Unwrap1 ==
  Estimated Angle : Inport
  Compare To Constant : simulink/Logic and Bit Operations/Compare To Constant  SystemSampleTime=-1  relop=>  const=180  LogicOutDataTypeMode=uint8  ZeroCross=off
  Compare To Constant1 : simulink/Logic and Bit Operations/Compare To Constant  SystemSampleTime=-1  relop=<  const=-180  LogicOutDataTypeMode=uint8  ZeroCross=off
  Compare To Zero : simulink/Logic and Bit Operations/Compare To Zero  SystemSampleTime=-1  relop=~=  LogicOutDataTypeMode=uint8  ZeroCross=off
  Difference : simulink/Discrete/Difference  SystemSampleTime=-1  ICPrevInput=0.0  OutMin=[]  OutMax=[]  OutDataType=sfix(16)  OutScaling=2^-10  DoSatur=off
  Discrete-Time Integrator : DiscreteIntegrator  gainval=1000  SampleTime=-1  OutDataType=sfix(16)  OutScaling=2^0  ICPrevOutput=DiscIntNeverNeededParam  ICPrevScaledInput=DiscIntNeverNeededParam
  Logical Operator : Logic  Orientation=up  Operator=NOR  AllPortsSameDT=off  OutDataTypeMode=boolean  OutDataTypeStr=boolean
  Lookup Table : Lookup  Orientation=left  InputValues=[-500 -195 195]  Table=[+360 0 -360]  LookUpMeth=Use Input Below  OutDataType=sfix(16)  OutScaling=2^0
  Merge : Merge  Inputs=3
  Sum2 : Sum  OutDataType=sfix(16)  OutScaling=2^0
  unwrap : Subsystem  TreatAsAtomicUnit=on
  unwrap1 : Subsystem  TreatAsAtomicUnit=on
  unwrap2 : Subsystem  TreatAsAtomicUnit=on
  unwrap angle : Outport
  Wrap : Outport  Port=2
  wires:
  Discrete-Time Integrator/1 -> unwrap angle/1, Lookup Table/1
  Estimated Angle/1 -> Difference/1
  unwrap1/1(Out1) -> Merge/3
  unwrap/1(Out1) -> Merge/2
  unwrap2/1(Out1) -> Merge/1
  Logical Operator/1 -> unwrap2/Enable
  Compare To Constant1/1 -> Logical Operator/2, unwrap1/Enable
  Compare To Constant/1 -> unwrap/Enable, Logical Operator/1
  Difference/1 -> unwrap2/1(In1), unwrap1/1(In1), Compare To Constant1/1, unwrap/1(In1), Compare To Constant/1
  Sum2/1 -> Discrete-Time Integrator/1
  Merge/1 -> Sum2/2
  Lookup Table/1 -> Sum2/1, Compare To Zero/1
  Compare To Zero/1 -> Wrap/1

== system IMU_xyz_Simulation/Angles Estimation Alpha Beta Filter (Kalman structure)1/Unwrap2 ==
  Estimated Angle : Inport
  Compare To Constant : simulink/Logic and Bit Operations/Compare To Constant  SystemSampleTime=-1  relop=>  const=180  LogicOutDataTypeMode=uint8  ZeroCross=off
  Compare To Constant1 : simulink/Logic and Bit Operations/Compare To Constant  SystemSampleTime=-1  relop=<  const=-180  LogicOutDataTypeMode=uint8  ZeroCross=off
  Compare To Zero : simulink/Logic and Bit Operations/Compare To Zero  SystemSampleTime=-1  relop=~=  LogicOutDataTypeMode=uint8  ZeroCross=off
  Difference : simulink/Discrete/Difference  SystemSampleTime=-1  ICPrevInput=0.0  OutMin=[]  OutMax=[]  OutDataType=sfix(16)  OutScaling=2^-10  DoSatur=off
  Discrete-Time Integrator : DiscreteIntegrator  gainval=1000  SampleTime=-1  OutDataType=sfix(16)  OutScaling=2^0  ICPrevOutput=DiscIntNeverNeededParam  ICPrevScaledInput=DiscIntNeverNeededParam
  Logical Operator : Logic  Orientation=up  Operator=NOR  AllPortsSameDT=off  OutDataTypeMode=boolean  OutDataTypeStr=boolean
  Lookup Table : Lookup  Orientation=left  InputValues=[-500 -195 195]  Table=[+360 0 -360]  LookUpMeth=Use Input Below  OutDataType=sfix(16)  OutScaling=2^0
  Merge : Merge  Inputs=3
  Sum2 : Sum  OutDataType=sfix(16)  OutScaling=2^0
  unwrap : Subsystem  TreatAsAtomicUnit=on
  unwrap1 : Subsystem  TreatAsAtomicUnit=on
  unwrap2 : Subsystem  TreatAsAtomicUnit=on
  unwrap angle : Outport
  Wrap : Outport  Port=2
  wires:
  Compare To Zero/1 -> Wrap/1
  Lookup Table/1 -> Compare To Zero/1, Sum2/1
  Merge/1 -> Sum2/2
  Sum2/1 -> Discrete-Time Integrator/1
  Difference/1 -> Compare To Constant/1, unwrap/1(In1), Compare To Constant1/1, unwrap1/1(In1), unwrap2/1(In1)
  Compare To Constant/1 -> Logical Operator/1, unwrap/Enable
  Compare To Constant1/1 -> unwrap1/Enable, Logical Operator/2
  Logical Operator/1 -> unwrap2/Enable
  unwrap2/1(Out1) -> Merge/1
  unwrap/1(Out1) -> Merge/2
  unwrap1/1(Out1) -> Merge/3
  Estimated Angle/1 -> Difference/1
  Discrete-Time Integrator/1 -> Lookup Table/1, unwrap angle/1

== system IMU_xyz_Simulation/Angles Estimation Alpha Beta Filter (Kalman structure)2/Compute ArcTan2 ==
  Force 1 : Inport
  Force 2 : Inport  Port=2
  Enable : EnablePort  StatesWhenEnabling=reset
  Gain1 : Gain  Gain=180/pi  ParameterDataType=sfix(16)  ParameterScaling=2^0  OutDataTypeMode=Specify via dialog  OutDataType=float('double')  OutDataTypeStr=float('double')
  Trigonometric Function1 : Trigonometry  Operator=atan2  OutputSignalType=real
  Degree : Outport
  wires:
  Trigonometric Function1/1 -> Gain1/1
  Gain1/1 -> Degree/1
  Force 1/1 -> Trigonometric Function1/1
  Force 2/1 -> Trigonometric Function1/2

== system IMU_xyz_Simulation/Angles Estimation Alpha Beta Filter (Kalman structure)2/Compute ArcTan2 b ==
  Force 1 : Inport
  Force 2 : Inport  Port=2
  Enable : EnablePort  StatesWhenEnabling=reset
  Gain1 : Gain  Gain=180/pi  ParameterDataType=sfix(16)  ParameterScaling=2^0  OutDataTypeMode=Specify via dialog  OutDataType=float('double')  OutDataTypeStr=float('double')
  Trigonometric Function1 : Trigonometry  Operator=atan2  OutputSignalType=real
  Degree : Outport
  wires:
  Force 2/1 -> Trigonometric Function1/2
  Force 1/1 -> Trigonometric Function1/1
  Gain1/1 -> Degree/1
  Trigonometric Function1/1 -> Gain1/1

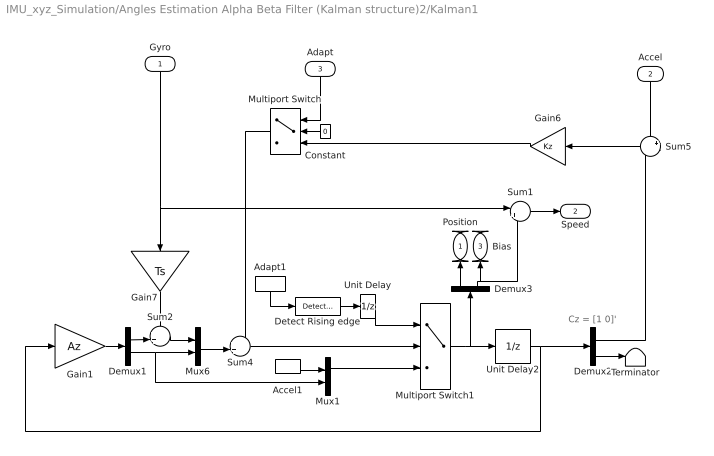
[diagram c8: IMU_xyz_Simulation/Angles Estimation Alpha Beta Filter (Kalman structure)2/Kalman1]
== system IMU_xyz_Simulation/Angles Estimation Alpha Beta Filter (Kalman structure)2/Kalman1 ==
  note: Cz = [1 0]'
  Gyro : Inport  Orientation=down
  Accel : Inport  Orientation=down  Port=2
  Adapt : Inport  Orientation=down  Port=3
  Accel1 : InportShadow  Port=2  LatchByCopyingInsideSignal=off
  Adapt1 : InportShadow  Orientation=down  Port=3  LatchByCopyingInsideSignal=off
  Constant : Constant  Orientation=left  Value=0  OutDataType=sfix(16)  OutScaling=2^0
  Demux1 : Demux  Outputs=2
  Demux2 : Demux  Outputs=2
  Demux3 : Demux  Orientation=up  Outputs=2
  Detect Rising edge : simulink/Logic and Bit Operations/Detect Increase  SystemSampleTime=-1  vinit=0
  Gain1 : Gain  Gain=Az  Multiplication=Matrix(K*u)  ParameterDataType=sfix(16)  ParameterScaling=2^0  OutDataType=sfix(16)  OutScaling=2^0
  Gain6 : Gain  Orientation=left  Gain=Kz  Multiplication=Matrix(K*u)  ParameterDataType=sfix(16)  ParameterScaling=2^0  OutDataType=sfix(16)  OutScaling=2^0
  Gain7 : Gain  Orientation=down  Gain=Ts  Multiplication=Matrix(K*u)  ParameterDataType=sfix(16)  ParameterScaling=2^0  OutDataType=sfix(16)  OutScaling=2^0
  Multiport Switch : MultiPortSwitch  Orientation=left  Inputs=2  zeroidx=on
  Multiport Switch1 : MultiPortSwitch  Inputs=2  zeroidx=on
  Mux1 : Mux  Inputs=2
  Mux6 : Mux  Inputs=2
  Sum1 : Sum  Inputs=|+-  OutDataType=sfix(16)  OutScaling=2^0
  Sum2 : Sum  Inputs=++|  OutDataType=sfix(16)  OutScaling=2^0
  Sum4 : Sum  Inputs=++|  OutDataType=sfix(16)  OutScaling=2^0
  Sum5 : Sum  Orientation=left  Inputs=+-  OutDataType=sfix(16)  OutScaling=2^0
  Terminator : Terminator
  Unit Delay : UnitDelay  SampleTime=-1
  Unit Delay2 : UnitDelay  SampleTime=-1
  Position : Outport  Orientation=up  OutDataType=sfix(16)  OutScaling=2^0
  Speed : Outport  Port=2  OutDataType=sfix(16)  OutScaling=2^0
  Bias : Outport  Orientation=up  Port=3  OutDataType=sfix(16)  OutScaling=2^0
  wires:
  Sum1/1 -> Speed/1
  Demux3/2 -> Sum1/2, Bias/1
  Demux3/1 -> Position/1
  Unit Delay2/1 -> Gain1/1, Demux2/1
  Unit Delay/1 -> Multiport Switch1/1
  Gyro/1 -> Sum1/1, Gain7/1
  Accel/1 -> Sum5/1
  Gain7/1 -> Sum2/1
  Sum5/1 -> Gain6/1
  Mux6/1 -> Sum4/2
  Demux1/2 -> Mux6/2, Mux1/2
  Sum2/1 -> Mux6/1
  Demux1/1 -> Sum2/2
  Gain1/1 -> Demux1/1
  Demux2/1 -> Sum5/2
  Multiport Switch/1 -> Sum4/1
  Adapt/1 -> Multiport Switch/1
  Gain6/1 -> Multiport Switch/3
  Constant/1 -> Multiport Switch/2
  Detect Rising edge/1 -> Unit Delay/1
  Multiport Switch1/1 -> Demux3/1, Unit Delay2/1
  Sum4/1 -> Multiport Switch1/2
  Adapt1/1 -> Detect Rising edge/1
  Accel1/1 -> Mux1/1
  Mux1/1 -> Multiport Switch1/3
  Demux2/2 -> Terminator/1

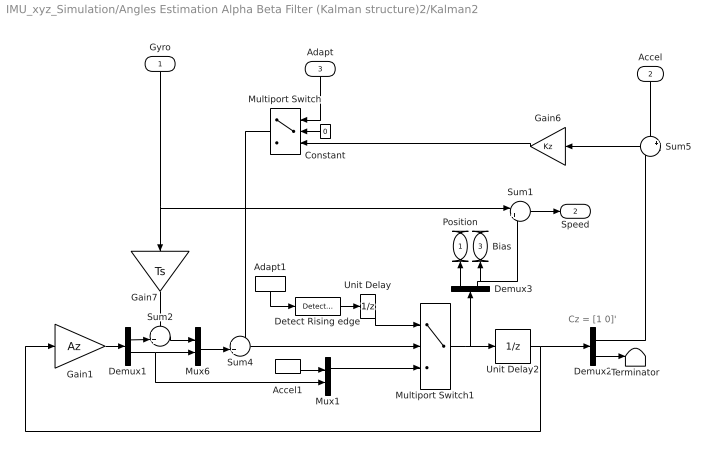
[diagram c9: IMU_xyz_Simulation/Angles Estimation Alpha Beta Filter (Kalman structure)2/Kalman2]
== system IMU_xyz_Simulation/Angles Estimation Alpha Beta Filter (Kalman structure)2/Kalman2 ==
  note: Cz = [1 0]'
  Gyro : Inport  Orientation=down
  Accel : Inport  Orientation=down  Port=2
  Adapt : Inport  Orientation=down  Port=3
  Accel1 : InportShadow  Port=2  LatchByCopyingInsideSignal=off
  Adapt1 : InportShadow  Orientation=down  Port=3  LatchByCopyingInsideSignal=off
  Constant : Constant  Orientation=left  Value=0  OutDataType=sfix(16)  OutScaling=2^0
  Demux1 : Demux  Outputs=2
  Demux2 : Demux  Outputs=2
  Demux3 : Demux  Orientation=up  Outputs=2
  Detect Rising edge : simulink/Logic and Bit Operations/Detect Increase  SystemSampleTime=-1  vinit=0
  Gain1 : Gain  Gain=Az  Multiplication=Matrix(K*u)  ParameterDataType=sfix(16)  ParameterScaling=2^0  OutDataType=sfix(16)  OutScaling=2^0
  Gain6 : Gain  Orientation=left  Gain=Kz  Multiplication=Matrix(K*u)  ParameterDataType=sfix(16)  ParameterScaling=2^0  OutDataType=sfix(16)  OutScaling=2^0
  Gain7 : Gain  Orientation=down  Gain=Ts  Multiplication=Matrix(K*u)  ParameterDataType=sfix(16)  ParameterScaling=2^0  OutDataType=sfix(16)  OutScaling=2^0
  Multiport Switch : MultiPortSwitch  Orientation=left  Inputs=2  zeroidx=on
  Multiport Switch1 : MultiPortSwitch  Inputs=2  zeroidx=on
  Mux1 : Mux  Inputs=2
  Mux6 : Mux  Inputs=2
  Sum1 : Sum  Inputs=|+-  OutDataType=sfix(16)  OutScaling=2^0
  Sum2 : Sum  Inputs=++|  OutDataType=sfix(16)  OutScaling=2^0
  Sum4 : Sum  Inputs=++|  OutDataType=sfix(16)  OutScaling=2^0
  Sum5 : Sum  Orientation=left  Inputs=+-  OutDataType=sfix(16)  OutScaling=2^0
  Terminator : Terminator
  Unit Delay : UnitDelay  SampleTime=-1
  Unit Delay2 : UnitDelay  SampleTime=-1
  Position : Outport  Orientation=up  OutDataType=sfix(16)  OutScaling=2^0
  Speed : Outport  Port=2  OutDataType=sfix(16)  OutScaling=2^0
  Bias : Outport  Orientation=up  Port=3  OutDataType=sfix(16)  OutScaling=2^0
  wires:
  Demux2/2 -> Terminator/1
  Mux1/1 -> Multiport Switch1/3
  Accel1/1 -> Mux1/1
  Adapt1/1 -> Detect Rising edge/1
  Sum4/1 -> Multiport Switch1/2
  Multiport Switch1/1 -> Unit Delay2/1, Demux3/1
  Detect Rising edge/1 -> Unit Delay/1
  Constant/1 -> Multiport Switch/2
  Gain6/1 -> Multiport Switch/3
  Adapt/1 -> Multiport Switch/1
  Multiport Switch/1 -> Sum4/1
  Demux2/1 -> Sum5/2
  Gain1/1 -> Demux1/1
  Demux1/1 -> Sum2/2
  Sum2/1 -> Mux6/1
  Demux1/2 -> Mux1/2, Mux6/2
  Mux6/1 -> Sum4/2
  Sum5/1 -> Gain6/1
  Gain7/1 -> Sum2/1
  Accel/1 -> Sum5/1
  Gyro/1 -> Gain7/1, Sum1/1
  Unit Delay/1 -> Multiport Switch1/1
  Unit Delay2/1 -> Demux2/1, Gain1/1
  Demux3/1 -> Position/1
  Demux3/2 -> Bias/1, Sum1/2
  Sum1/1 -> Speed/1

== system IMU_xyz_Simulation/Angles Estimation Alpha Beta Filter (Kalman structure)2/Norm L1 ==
  Accel Y : Inport
  Accel Z : Inport  Port=2
  Accel X : Inport  Port=3
  Abs : Abs
  Abs1 : Abs
  Abs2 : Abs
  Sum1 : Sum  OutDataType=sfix(16)  OutScaling=2^0
  Sum3 : Sum  OutDataType=sfix(16)  OutScaling=2^0
  abs(Y)+abs(Z) : Outport
  abs(X)+abs(Z) : Outport  Port=2
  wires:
  Abs/1 -> Sum3/1
  Abs1/1 -> Sum1/1, Sum3/2
  Accel Y/1 -> Abs/1
  Accel Z/1 -> Abs1/1
  Sum3/1 -> abs(Y)+abs(Z)/1
  Abs2/1 -> Sum1/2
  Accel X/1 -> Abs2/1
  Sum1/1 -> abs(X)+abs(Z)/1

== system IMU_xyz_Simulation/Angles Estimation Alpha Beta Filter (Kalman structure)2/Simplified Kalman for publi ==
  note: Cz = [1 0]'
  Gyro : Inport  Orientation=down
  Accel : Inport  Orientation=down  Port=2
  Demux1 : Demux  Outputs=2
  Demux2 : Demux  Outputs=2
  Gain1 : Gain  Gain=Az  Multiplication=Matrix(K*u)  ParameterDataType=sfix(16)  ParameterScaling=2^0  OutDataType=sfix(16)  OutScaling=2^0
  Gain6 : Gain  Orientation=left  Gain=Kz  Multiplication=Matrix(K*u)  ParameterDataType=sfix(16)  ParameterScaling=2^0  OutDataType=sfix(16)  OutScaling=2^0
  Gain7 : Gain  Orientation=down  Gain=Ts  Multiplication=Matrix(K*u)  ParameterDataType=sfix(16)  ParameterScaling=2^0  OutDataType=sfix(16)  OutScaling=2^0
  Mux6 : Mux  Inputs=2
  Sum2 : Sum  Inputs=++|  OutDataType=sfix(16)  OutScaling=2^0
  Sum4 : Sum  Inputs=++|  OutDataType=sfix(16)  OutScaling=2^0
  Sum5 : Sum  Orientation=left  Inputs=+-  OutDataType=sfix(16)  OutScaling=2^0
  Terminator : Terminator
  Unit Delay2 : UnitDelay  SampleTime=-1
  Angle Estimation : Outport  OutDataType=sfix(16)  OutScaling=2^0
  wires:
  Demux2/2 -> Terminator/1
  Sum4/1 -> Unit Delay2/1
  Demux2/1 -> Sum5/2, Angle Estimation/1
  Gain1/1 -> Demux1/1
  Demux1/1 -> Sum2/2
  Sum2/1 -> Mux6/1  "Angle Estimation"
  Demux1/2 -> Mux6/2  "Gyro Bias"
  Mux6/1 -> Sum4/2
  Sum5/1 -> Gain6/1
  Gain7/1 -> Sum2/1
  Accel/1 -> Sum5/1
  Gyro/1 -> Gain7/1
  Unit Delay2/1 -> Demux2/1, Gain1/1
  Gain6/1 -> Sum4/1

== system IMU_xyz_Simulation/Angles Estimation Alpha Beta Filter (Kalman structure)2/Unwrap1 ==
  Estimated Angle : Inport
  Compare To Constant : simulink/Logic and Bit Operations/Compare To Constant  SystemSampleTime=-1  relop=>  const=180  LogicOutDataTypeMode=uint8  ZeroCross=off
  Compare To Constant1 : simulink/Logic and Bit Operations/Compare To Constant  SystemSampleTime=-1  relop=<  const=-180  LogicOutDataTypeMode=uint8  ZeroCross=off
  Compare To Zero : simulink/Logic and Bit Operations/Compare To Zero  SystemSampleTime=-1  relop=~=  LogicOutDataTypeMode=uint8  ZeroCross=off
  Difference : simulink/Discrete/Difference  SystemSampleTime=-1  ICPrevInput=0.0  OutMin=[]  OutMax=[]  OutDataType=sfix(16)  OutScaling=2^-10  DoSatur=off
  Discrete-Time Integrator : DiscreteIntegrator  gainval=1000  SampleTime=-1  OutDataType=sfix(16)  OutScaling=2^0  ICPrevOutput=DiscIntNeverNeededParam  ICPrevScaledInput=DiscIntNeverNeededParam
  Logical Operator : Logic  Orientation=up  Operator=NOR  AllPortsSameDT=off  OutDataTypeMode=boolean  OutDataTypeStr=boolean
  Lookup Table : Lookup  Orientation=left  InputValues=[-500 -195 195]  Table=[+360 0 -360]  LookUpMeth=Use Input Below  OutDataType=sfix(16)  OutScaling=2^0
  Merge : Merge  Inputs=3
  Sum2 : Sum  OutDataType=sfix(16)  OutScaling=2^0
  unwrap : Subsystem  TreatAsAtomicUnit=on
  unwrap1 : Subsystem  TreatAsAtomicUnit=on
  unwrap2 : Subsystem  TreatAsAtomicUnit=on
  unwrap angle : Outport
  Wrap : Outport  Port=2
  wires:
  Compare To Zero/1 -> Wrap/1
  Lookup Table/1 -> Compare To Zero/1, Sum2/1
  Merge/1 -> Sum2/2
  Sum2/1 -> Discrete-Time Integrator/1
  Difference/1 -> Compare To Constant/1, unwrap/1(In1), Compare To Constant1/1, unwrap1/1(In1), unwrap2/1(In1)
  Compare To Constant/1 -> Logical Operator/1, unwrap/Enable
  Compare To Constant1/1 -> unwrap1/Enable, Logical Operator/2
  Logical Operator/1 -> unwrap2/Enable
  unwrap2/1(Out1) -> Merge/1
  unwrap/1(Out1) -> Merge/2
  unwrap1/1(Out1) -> Merge/3
  Estimated Angle/1 -> Difference/1
  Discrete-Time Integrator/1 -> Lookup Table/1, unwrap angle/1

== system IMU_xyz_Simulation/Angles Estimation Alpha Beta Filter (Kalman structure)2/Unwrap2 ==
  Estimated Angle : Inport
  Compare To Constant : simulink/Logic and Bit Operations/Compare To Constant  SystemSampleTime=-1  relop=>  const=180  LogicOutDataTypeMode=uint8  ZeroCross=off
  Compare To Constant1 : simulink/Logic and Bit Operations/Compare To Constant  SystemSampleTime=-1  relop=<  const=-180  LogicOutDataTypeMode=uint8  ZeroCross=off
  Compare To Zero : simulink/Logic and Bit Operations/Compare To Zero  SystemSampleTime=-1  relop=~=  LogicOutDataTypeMode=uint8  ZeroCross=off
  Difference : simulink/Discrete/Difference  SystemSampleTime=-1  ICPrevInput=0.0  OutMin=[]  OutMax=[]  OutDataType=sfix(16)  OutScaling=2^-10  DoSatur=off
  Discrete-Time Integrator : DiscreteIntegrator  gainval=1000  SampleTime=-1  OutDataType=sfix(16)  OutScaling=2^0  ICPrevOutput=DiscIntNeverNeededParam  ICPrevScaledInput=DiscIntNeverNeededParam
  Logical Operator : Logic  Orientation=up  Operator=NOR  AllPortsSameDT=off  OutDataTypeMode=boolean  OutDataTypeStr=boolean
  Lookup Table : Lookup  Orientation=left  InputValues=[-500 -195 195]  Table=[+360 0 -360]  LookUpMeth=Use Input Below  OutDataType=sfix(16)  OutScaling=2^0
  Merge : Merge  Inputs=3
  Sum2 : Sum  OutDataType=sfix(16)  OutScaling=2^0
  unwrap : Subsystem  TreatAsAtomicUnit=on
  unwrap1 : Subsystem  TreatAsAtomicUnit=on
  unwrap2 : Subsystem  TreatAsAtomicUnit=on
  unwrap angle : Outport
  Wrap : Outport  Port=2
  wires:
  Discrete-Time Integrator/1 -> unwrap angle/1, Lookup Table/1
  Estimated Angle/1 -> Difference/1
  unwrap1/1(Out1) -> Merge/3
  unwrap/1(Out1) -> Merge/2
  unwrap2/1(Out1) -> Merge/1
  Logical Operator/1 -> unwrap2/Enable
  Compare To Constant1/1 -> Logical Operator/2, unwrap1/Enable
  Compare To Constant/1 -> unwrap/Enable, Logical Operator/1
  Difference/1 -> unwrap2/1(In1), unwrap1/1(In1), Compare To Constant1/1, unwrap/1(In1), Compare To Constant/1
  Sum2/1 -> Discrete-Time Integrator/1
  Merge/1 -> Sum2/2
  Lookup Table/1 -> Sum2/1, Compare To Zero/1
  Compare To Zero/1 -> Wrap/1

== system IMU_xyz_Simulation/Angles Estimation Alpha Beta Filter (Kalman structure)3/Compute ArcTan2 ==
  Force 1 : Inport
  Force 2 : Inport  Port=2
  Enable : EnablePort  StatesWhenEnabling=reset
  Gain1 : Gain  Gain=180/pi  ParameterDataType=sfix(16)  ParameterScaling=2^0  OutDataTypeMode=Specify via dialog  OutDataType=float('double')  OutDataTypeStr=float('double')
  Trigonometric Function1 : Trigonometry  Operator=atan2  OutputSignalType=real
  Degree : Outport
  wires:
  Force 2/1 -> Trigonometric Function1/2
  Force 1/1 -> Trigonometric Function1/1
  Gain1/1 -> Degree/1
  Trigonometric Function1/1 -> Gain1/1

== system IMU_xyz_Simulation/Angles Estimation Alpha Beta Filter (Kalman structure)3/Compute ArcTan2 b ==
  Force 1 : Inport
  Force 2 : Inport  Port=2
  Enable : EnablePort  StatesWhenEnabling=reset
  Gain1 : Gain  Gain=180/pi  ParameterDataType=sfix(16)  ParameterScaling=2^0  OutDataTypeMode=Specify via dialog  OutDataType=float('double')  OutDataTypeStr=float('double')
  Trigonometric Function1 : Trigonometry  Operator=atan2  OutputSignalType=real
  Degree : Outport
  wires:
  Trigonometric Function1/1 -> Gain1/1
  Gain1/1 -> Degree/1
  Force 1/1 -> Trigonometric Function1/1
  Force 2/1 -> Trigonometric Function1/2
